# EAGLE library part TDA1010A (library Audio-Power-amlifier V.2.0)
The TDA1010A is a monolithic integrated class-B audio amplifier circuit in a 9-lead single in-line (SIL) plastic package. The device is primarily developed as a 6 W car radio amplifier for use with 4 Wand 2 Wload impedances. The wide supply voltage range and the flexibility of the IC make it an attractive proposition for record players and tape recorders with output powers up to 10 W.
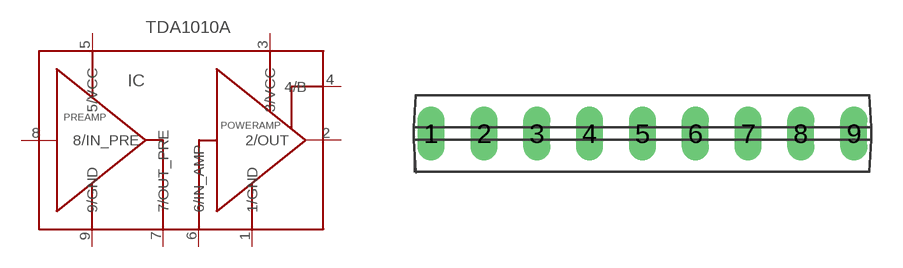
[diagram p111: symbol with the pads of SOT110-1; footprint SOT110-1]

Designator prefix IC

## TDA1010A  [SOT110-1]
1  1/GND  pwr
2  2/OUT  out
3  3/VCC  pwr
4  4/B
5  5/VCC  pwr
6  6/IN_AMP  in
7  7/OUT_PRE  out
8  8/IN_PRE  in
9  9/GND  pwr

## Footprint SOT110-1 (pad centres in mm)
SIL9MPF: plastic single in-line medium power package with fin; 9 leads
drill 0.8 long: 1 -10.16,0; 2 -7.62,0; 3 -5.08,0; 4 -2.54,0; 5 0,0; 6 2.54,0; 7 5.08,0; 8 7.62,0; 9 10.16,0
